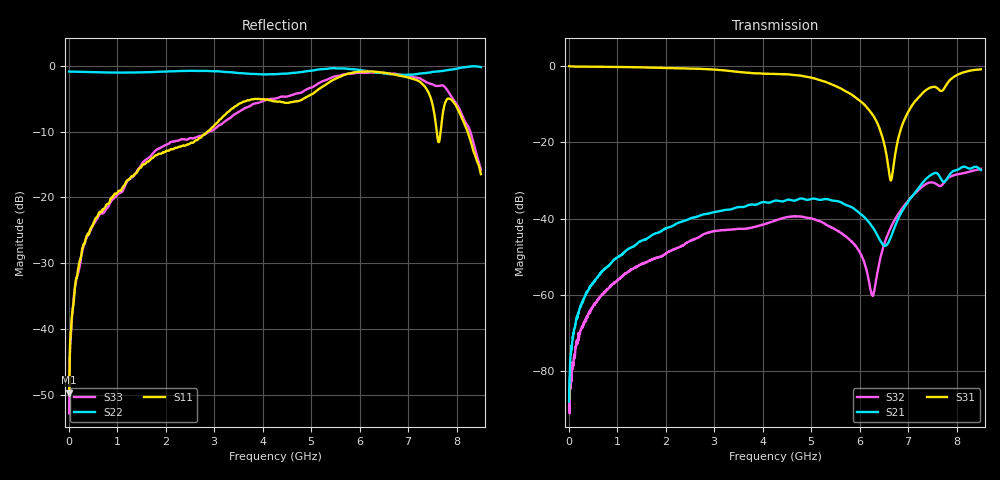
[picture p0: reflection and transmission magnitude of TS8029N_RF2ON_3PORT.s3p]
!Created with skrf (http://scikit-rf.org).
# GHz S RI R 50.0
!freq ReS11 ImS11 ReS12 ImS12 ReS13 ImS13
! ReS21 ImS21 ReS22 ImS22 ReS23 ImS23
! ReS31 ImS31 ReS32 ImS32 ReS33 ImS33
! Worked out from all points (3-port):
!   1601 points, 10 MHz to 8.5 GHz, reference 50 ohm
!   strongest paths, dB at 10 MHz, 2.132 GHz, 4.255 GHz, 6.378 GHz, 8.5 GHz:
!     S31: 0.0, -0.6, -2.1, -15.3, -0.9
!     S21: -87.9, -42.0, -35.3, -44.6, -27.3
!     S32: -89.7, -48.3, -40.5, -53.5, -26.9
!   lowest |S11| = -49.7 dB at 10 MHz (marker M1), VSWR 1.01, Z = 50.1 + j0.32 ohm
!   |S11| at or under -10 dB: start of sweep to 2.862 GHz; 7.59 GHz to 7.67 GHz (80.58 MHz wide, 1.06 % of centre); 8.226 GHz to end of sweep
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0.01  0.00074 0.0032  2.7e-05 4.91e-05  0.9944 -0.00869
      1.63e-05 3.67e-05  -0.9055 0.00342  4.45e-05 -1.92e-06
      0.9943 -0.00873  2.66e-05 1.9e-05  0.00197 0.00117
0.1479625  0.00839 -0.022  7.96e-05 0.000436  0.9805 -0.0569
           6.78e-05 0.00044  -0.9012 0.0353  6.48e-05 -0.000176
           0.9804 -0.057  4.6e-05 -0.000197  0.00702 -0.0213
0.625525  -0.0033 -0.0762  -0.000122 0.00181  0.9489 -0.2268
          -0.000111 0.0018  -0.8789 0.1566  -0.000544 -0.000758
          0.9489 -0.2267  -0.000534 -0.000716  -0.00937 -0.0721
4.255  -0.5371 0.0265  0.00876 0.0149  -0.0753 -0.7839
       0.00875 0.0148  -0.3149 0.8032  -0.000297 0.00939
       -0.0762 -0.7822  -0.000308 0.00938  -0.563 -0.0114
5.671769  -0.5438 0.6537  0.0136 0.00775  -0.3496 -0.3303
          0.0136 0.00774  -0.0127 0.9543  0.00446 0.00414
          -0.3497 -0.3303  0.00454 0.00407  -0.551 0.6605
6.266069  -0.2284 0.8754  0.00673 0.00393  -0.2083 -0.0975
          0.00671 0.00392  0.0276 0.9025  -0.000251 0.00096
          -0.2084 -0.0975  -0.000243 0.000943  -0.3918 0.7978
6.642812  0.0444 0.8664  -0.00142 0.00552  -0.00336 -0.0313
          -0.00146 0.00554  0.146 0.8502  -0.00733 0.00223
          -0.00346 -0.0313  -0.00736 0.0022  0.0582 0.869
7.157519  0.4884 0.6133  -0.00749 0.0212  0.2369 -0.2614
          -0.00751 0.0212  0.3738 0.7769  -0.0133 0.0174
          0.2369 -0.2614  -0.0133 0.0174  0.5733 0.5786
7.555487  0.3768 0.1228  0.00889 0.0388  0.1203 -0.5183
          0.00894 0.0386  0.4996 0.7506  8.72e-05 0.029
          0.1186 -0.5185  -1.87e-05 0.029  0.5523 0.4409
8.5  0.102 0.1104  0.0232 0.0366  -0.2522 -0.869
     0.0232 0.0366  0.5174 0.8282  0.0186 0.041
     -0.2526 -0.8683  0.0185 0.0409  0.161 -0.00794
